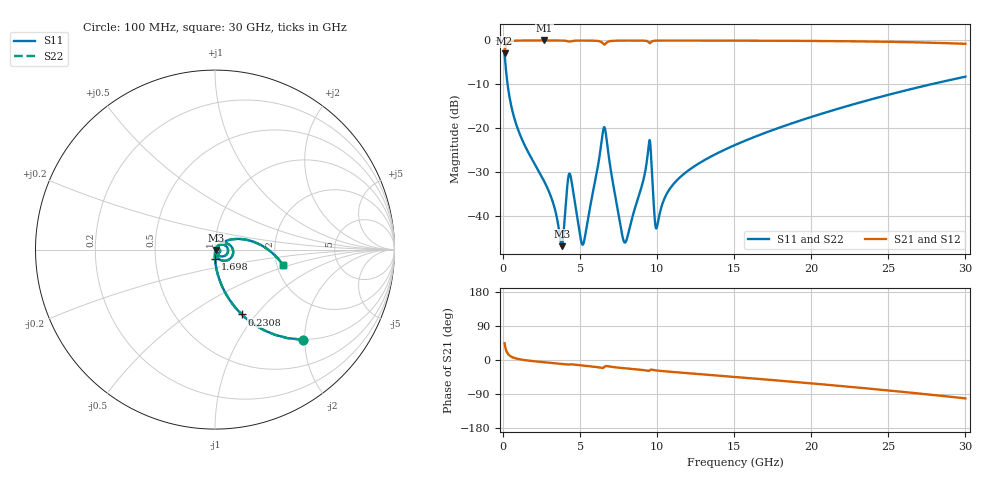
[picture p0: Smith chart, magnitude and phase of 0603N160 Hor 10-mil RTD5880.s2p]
# GHz S MA R 50
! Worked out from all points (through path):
!   3201 points, 100 MHz to 30 GHz, reference 50 ohm
!   highest |S21| = -0.02 dB at 2.679 GHz (marker M1); lowest = -2.9 dB at 100 MHz (marker M2)
!   group delay of S21, straight-line fit = 9.61 ps
!   lowest |S11| = -46.8 dB at 3.809 GHz (marker M3), VSWR 1.01, Z = 50.4 - j0.245 ohm
!   |S11| at or under -10 dB: 293.3 MHz to 27.76 GHz (27.46 GHz wide, 196 % of centre)
!   |S22| runs from -46.8 to -3.1 dB; largest |S21 - S12| = 0
!   S11 on the Smith chart (normalised r, x): 100 MHz: 0.99, -1.95; 230.8 MHz: 0.99, -0.84; 1.698 GHz: 0.99, -0.10; 30 GHz: 2.16, -0.42
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0.1  0.7002 -45.8  0.7137 44.2  0.7137 44.2  0.7002 -45.8
0.2308125  0.3905 -67.6  0.9202 22.3  0.9202 22.3  0.3905 -67.6
0.735375  0.1294 -84.3  0.9908 5.4  0.9908 5.4  0.1294 -84.3
1.697781  0.05086 -90.5  0.9975 -1.8  0.9975 -1.8  0.05086 -90.5
2.678875  0.02474 -92.5  0.9981 -6.0  0.9981 -6.0  0.02474 -92.5
3.809469  0.004566 -32.2  0.9957 -10.5  0.9957 -10.5  0.004566 -32.2
4.332719  0.03033 -30.0  0.9711 -11.5  0.9711 -11.5  0.03033 -30.0
5.089563  0.005024 -28.0  0.995 -14.1  0.995 -14.1  0.005024 -28.0
5.323156  0.005977 24.2  0.9953 -15.0  0.9953 -15.0  0.005977 24.2
6.556531  0.1031 -11.1  0.8977 -19.0  0.8977 -19.0  0.1031 -11.1
7.855313  0.005103 -25.7  0.9948 -21.7  0.9948 -21.7  0.005103 -25.7
9.004594  0.02219 48.8  0.9939 -26.1  0.9939 -26.1  0.02219 48.8
9.462438  0.06687 14.7  0.9502 -28.8  0.9502 -28.8  0.06687 14.7
9.59325  0.05256 -46.6  0.9507 -25.4  0.9507 -25.4  0.05256 -46.6
9.873563  0.008113 -31.5  0.9918 -27.2  0.9918 -27.2  0.008113 -31.5
10.06978  0.00891 24.1  0.9944 -28.2  0.9944 -28.2  0.00891 24.1
10.54631  0.01697 46.1  0.9956 -30.0  0.9956 -30.0  0.01697 46.1
11.34988  0.02637 49.1  0.9958 -32.7  0.9958 -32.7  0.02637 49.1
15.05  0.06458 41.6  0.9936 -44.8  0.9936 -44.8  0.06458 41.6
20.03956  0.1353 26.1  0.9855 -61.8  0.9855 -61.8  0.1353 26.1
25.01978  0.241 8.1  0.964 -80.5  0.964 -80.5  0.241 8.1
30  0.3865 -12.4  0.9142 -101.3  0.9142 -101.3  0.3865 -12.4
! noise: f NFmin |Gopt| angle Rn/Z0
0.1  0.0003079  0.9225  0.4615  0.00088
3.417  0.004071  0.8114  9.516  0.00447
6.743  0.02758  0.9414  18.69  0.1024
10.06  0.01097  0.798  27.73  0.01061
13.39  0.01058  0.7335  36.55  0.007161
16.7  0.01254  0.7242  45.17  0.007729
20.03  0.01471  0.7217  53.59  0.008403
23.35  0.01707  0.7238  61.75  0.009116
26.67  0.0197  0.7294  69.7  0.009875
30  0.02267  0.7379  77.42  0.01069
